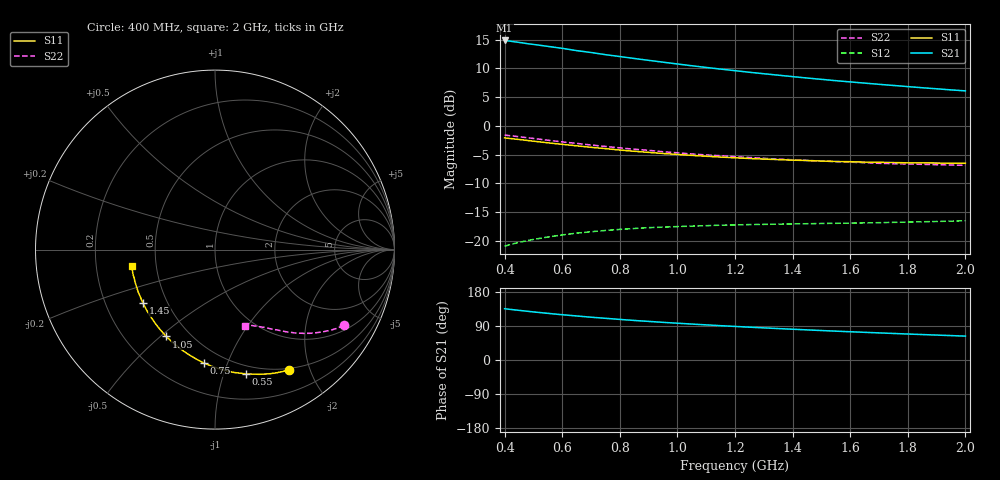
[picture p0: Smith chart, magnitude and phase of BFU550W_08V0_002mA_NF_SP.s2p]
! Filename:  P:\Prog\Test\Noise\ATS_data\Testdata_Net\06 Compressed Noise after Statistics\BFU550W_APM2013_11_D05_08p0V_002mA_NF_CM01_D.sf
! Date/Time: Tue 26/Mar/2013 16:25:23
! BFU550W_APM2013_11_D05_08p0V_1to35mA_NF_CM01_Bias2_R.sf
! Noise Parameter Data File
! BFU550W_APM2013_11_D05_08p0V_1to35mA_NF_CM01
! Date/time: Mon Mar 25 14:39:45 2013
! VAR V_out= 8.000000
! VAR I_out= 1.995000
! VAR V_in= 0.788900
! VAR I_in= 0.019600
! Device data file deembeded for feedlines and parallel
! Original file: \06 Compressed Noise after Statistics\BFU550W_APM2013_11_D05_08p0V_002mA_NF_CM01_R.sf
! Feed-files: PR019V01_070313_Feed1.s2p, PR019V01_070313_Feed2.s2p
! Parallel-file: PR019V01_070313_Par.s2p
# MHz S MA R 50
!  Freq-MHz  S11-mag  S11-arg  S21-mag  S21-arg  S12-mag  S12-arg  S22-mag  S22-arg
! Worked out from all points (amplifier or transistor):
!   37 points, 400 MHz to 2 GHz, reference 50 ohm
!   highest |S21| = 14.9 dB at 400 MHz (marker M1)
!   |S21| within 3 dB of that: start of sweep to 830.3 MHz
!   unconditionally stable (mu >= 1): nowhere
!   at 500 MHz: K = 0.28, MSG = 17.0 dB, |S12| = -19.7 dB
!   at 1.1 GHz: K = 0.59, MSG = 13.8 dB, |S12| = -17.3 dB
!   at 2 GHz: K = 0.96, MSG = 11.3 dB, |S12| = -16.5 dB
!   lowest NFmin = 0.43 dB at 420 MHz
!   S11 on the Smith chart (normalised r, x): 400 MHz: 0.48, -1.68; 550 MHz: 0.42, -1.19; 750 MHz: 0.39, -0.83; 1.05 GHz: 0.37, -0.52; 1.45 GHz: 0.36, -0.29; 2 GHz: 0.36, -0.09
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400  0.7876 -58.5  5.534 135.3  0.09009 57.6  0.8326 -30.4
420  0.7765 -61.1  5.455 133.5  0.09302 56.5  0.8219 -31.5
460  0.7574 -65.9  5.281 130.2  0.09836 54.3  0.8003 -33.6
500  0.7369 -70.6  5.113 126.9  0.1031 52.3  0.7782 -35.5
550  0.7131 -76.1  4.917 123.1  0.1082 50.1  0.7511 -37.7
600  0.6917 -81.5  4.726 119.5  0.1128 48.1  0.7264 -39.6
650  0.6717 -86.3  4.515 116.2  0.117 46.4  0.7052 -41.4
700  0.6515 -91.3  4.349 112.9  0.1202 44.7  0.6826 -43.2
750  0.635 -95.7  4.165 110.0  0.1234 43.4  0.6633 -44.6
800  0.6171 -100.1  4.011 107.1  0.126 42.1  0.6447 -46.1
850  0.602 -104.3  3.858 104.4  0.1283 41.1  0.6274 -47.3
950  0.576 -112.1  3.583 99.4  0.1318 39.3  0.5966 -49.8
1050  0.5549 -119.3  3.335 94.8  0.1346 38.1  0.5706 -51.9
1150  0.5361 -126.1  3.119 90.6  0.1372 37.1  0.5509 -53.8
1200  0.5285 -129.1  3.023 88.6  0.1378 36.9  0.5399 -54.9
1250  0.5209 -132.3  2.929 86.6  0.1389 36.6  0.5316 -55.6
1350  0.5095 -138.0  2.761 83.0  0.14 36.6  0.5141 -57.5
1450  0.5002 -143.5  2.609 79.5  0.1412 36.7  0.501 -59.2
1500  0.4951 -146.1  2.541 77.8  0.1419 36.8  0.4955 -60.1
1600  0.4886 -151.2  2.414 74.6  0.1429 37.4  0.4841 -61.9
1750  0.4807 -158.1  2.248 70.0  0.1451 38.7  0.4697 -64.2
2000  0.4738 -168.8  2.017 63.0  0.1499 41.5  0.4543 -68.6
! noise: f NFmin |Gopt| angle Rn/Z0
400  0.48  0.509  32.07  0.1719
460  0.4894  0.5043  36.01  0.1755
600  0.5361  0.4852  44.65  0.1842
800  0.5997  0.4718  62.01  0.156
1000  0.6904  0.478  74.15  0.1535
1200  0.7504  0.4738  89.46  0.134
1400  0.7816  0.4576  104.8  0.1156
1600  0.7357  0.4423  124.5  0.0882
1800  0.9401  0.4629  133.3  0.0804
2000  0.9664  0.4338  149.9  0.0745
